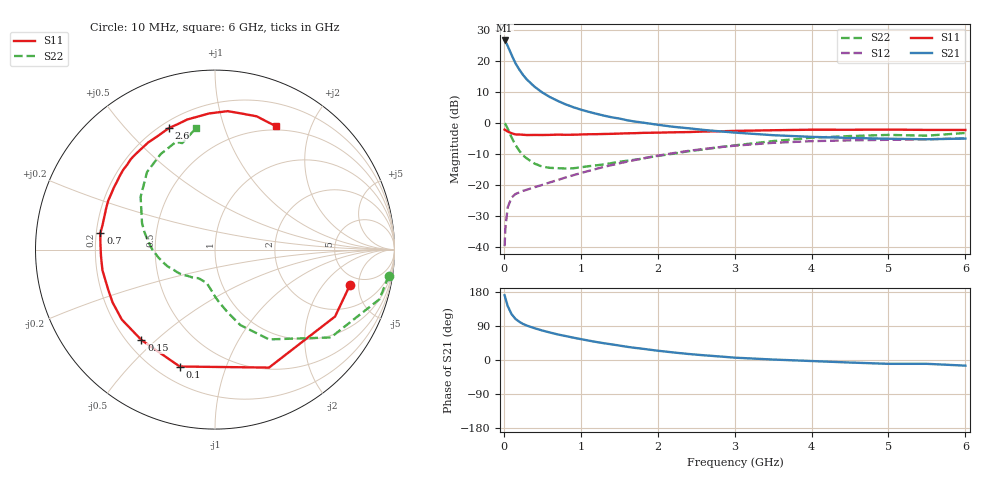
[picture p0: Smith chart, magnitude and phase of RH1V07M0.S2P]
! SIEMENS Small Signal Semiconductors
! BFR106
! Si NPN RF Bipolar Junction Transistor in SOT23
! VCE = 1 V  IC = 7 mA
! Common Emitter S-Parameters:  August  1996
# GHz  S  MA  R  50
!  f  S11  S21  S12  S22
! GHz  MAG  ANG  MAG  ANG  MAG  ANG  MAG  ANG
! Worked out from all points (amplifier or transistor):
!   36 points, 10 MHz to 6 GHz, reference 50 ohm
!   highest |S21| = 26.5 dB at 10 MHz (marker M1)
!   |S21| within 3 dB of that: start of sweep to 71.72 MHz
!   unconditionally stable (mu >= 1): 518.3 MHz to 2.927 GHz; 3.659 GHz to end of sweep
!   at 250 MHz: K = 0.61, MSG = 18.7 dB, |S12| = -21.9 dB
!   at 1.4 GHz: K = 1.16, MAG = 5.3 dB, |S12| = -13.6 dB
!   at 6 GHz: K = 1.03, MAG = -1.1 dB, |S12| = -5.0 dB
!   S11 on the Smith chart (normalised r, x): 10 MHz: 3.91, -3.92; 100 MHz: 0.29, -0.70; 150 MHz: 0.26, -0.45; 700 MHz: 0.22, +0.07; 2.6 GHz: 0.23, +0.66; 6 GHz: 0.45, +1.51
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0.01  0.7772 -14.8  21.22 170.8  0.0103 84.2  0.9793 -8.5
0.02  0.7659 -29.1  20.58 163.3  0.0201 75.5  0.957 -16.8
0.05  0.723 -65.4  17.35 142.3  0.0433 59.2  0.8098 -37.2
0.1  0.6804 -106.8  12.46 121.2  0.0625 44.6  0.5836 -59.0
0.15  0.6495 -129.1  9.165 108.7  0.0711 37.9  0.4429 -71.5
0.2  0.6493 -143.1  7.244 101.0  0.0756 36.4  0.3565 -78.6
0.25  0.6421 -152.7  5.896 95.0  0.0802 36.3  0.2981 -85.0
0.3  0.6356 -159.3  4.971 90.8  0.0836 37.4  0.2658 -89.4
0.4  0.6376 -169.6  3.81 83.8  0.0918 39.8  0.2203 -96.6
0.5  0.6363 -176.8  3.08 77.8  0.1001 42.8  0.1967 -102.4
0.6  0.6392 177.0  2.598 72.5  0.1097 45.1  0.1881 -107.3
0.7  0.6451 171.9  2.258 67.5  0.1198 47.5  0.1859 -112.2
0.9  0.643 163.7  1.791 59.1  0.143 50.4  0.1851 -120.7
1.1  0.6545 155.4  1.507 51.3  0.1676 52.2  0.1999 -129.1
1.3  0.661 148.5  1.307 44.3  0.1949 52.3  0.2137 -137.3
1.6  0.6775 139.1  1.101 34.9  0.2367 51.2  0.2448 -148.9
2.2  0.7033 122.0  0.864 20.0  0.3245 44.8  0.3172 -171.7
2.6  0.724 110.9  0.767 12.5  0.3793 38.7  0.373 173.4
3.5  0.7592 92.5  0.632 1.2  0.476 23.4  0.5077 144.7
4.5  0.7727 78.1  0.571 -6.7  0.5219 7.6  0.6123 119.6
5.5  0.7687 67.4  0.544 -10.1  0.5418 -1.7  0.6207 107.1
6  0.7672 63.7  0.557 -14.9  0.564 -8.6  0.6861 98.7
